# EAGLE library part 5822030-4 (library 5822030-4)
Body Features: Retention Post Location Center | Latch Plating Material Nickel | Connector Profile Standard | Latch Material Brass | Configuration Features: Number of Positions 80 | Module Orientation Vertical | Number of Keys 1 | Number of Rows 1 | Contact Features: Contact Mating Area Plating Material Thickness 200 MICIN | Contact Current Rating (Max) 1 AMP | Contact Mating Area Plating Material Tin | PCB Contact Termination Area Plating Material Tin | Memory Socket Type Memory Card | Contact Base Material Source: Datasheet
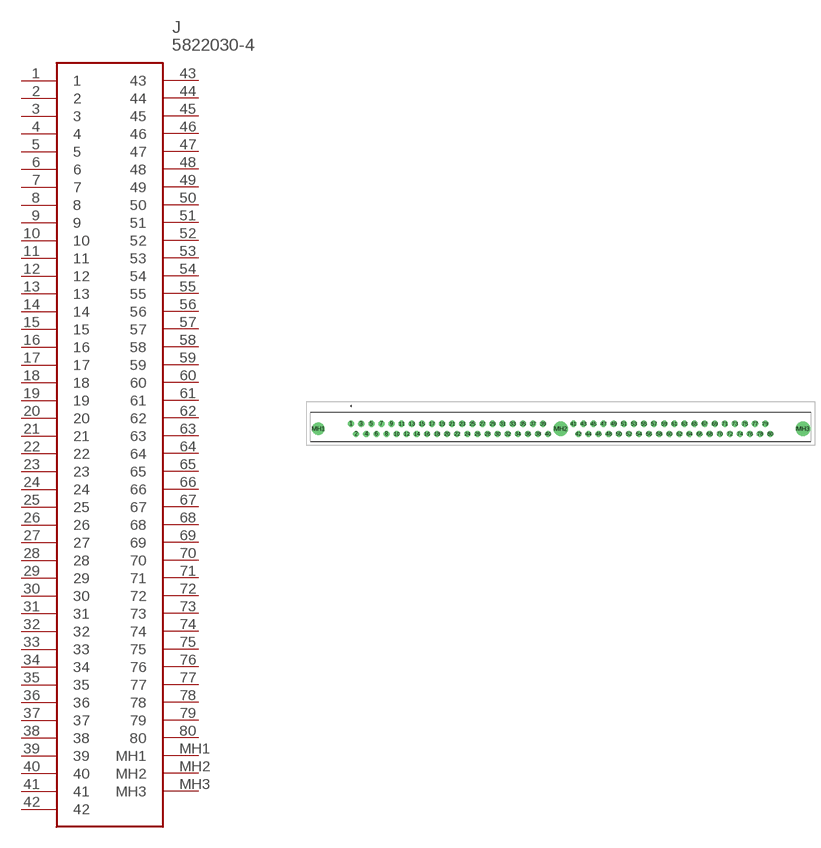
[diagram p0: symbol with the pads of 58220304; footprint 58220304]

Designator prefix J

## 5822030-4 (Description: Body Features: Retention Post Location Center | Latch Plating Material Nickel | Connector Profile Standard | Latch Material Brass | Configuration Features: Number of Positions 80 | Module Orientation Vertical | Number of Keys 1 | Number of Rows 1 | Contact Features: Contact Mating Area Plating Material Thickness 200 MICIN | Contact Current Rating (Max) 1 AMP | Contact Mating Area Plating Material Tin | PCB Contact Termination Area Plating Material Tin | Memory Socket Type Memory Card | Contact Base Material; Height: 14.61mm; Manufacturer_Name: TE Connectivity; Manufacturer_Part_Number: 5822030-4; Mouser_Part_Number: 571-58220304; Mouser_Price-Stock: https://www.mouser.co.uk/ProductDetail/TE-Connectivity/5822030-4?qs=VZ9FDhhp7SlQjd0753bE2g%3D%3D)  [58220304]
1  1
2  2
3  3
4  4
5  5
6  6
7  7
8  8
9  9
10  10
11  11
12  12
13  13
14  14
15  15
16  16
17  17
18  18
19  19
20  20
21  21
22  22
23  23
24  24
25  25
26  26
27  27
28  28
29  29
30  30
31  31
32  32
33  33
34  34
35  35
36  36
37  37
38  38
39  39
40  40
41  41
42  42
43  43
44  44
45  45
46  46
47  47
48  48
49  49
50  50
51  51
52  52
53  53
54  54
55  55
56  56
57  57
58  58
59  59
60  60
61  61
62  62
63  63
64  64
65  65
66  66
67  67
68  68
69  69
70  70
71  71
72  72
73  73
74  74
75  75
76  76
77  77
78  78
79  79
80  80
MH1  MH1
MH2  MH2
MH3  MH3

## Footprint 58220304 (pad centres in mm)
5822030-4-2
drill 1.02 pad 1.53: 1 0,0; 2 1.27,-2.54; 3 2.54,0; 4 3.81,-2.54; 5 5.08,0; 6 6.35,-2.54; 7 7.62,0; 8 8.89,-2.54; 9 10.16,0; 10 11.43,-2.54; 11 12.7,0; 12 13.97,-2.54; 13 15.24,0; 14 16.51,-2.54; 15 17.78,0; 16 19.05,-2.54; 17 20.32,0; 18 21.59,-2.54; 19 22.86,0; 20 24.13,-2.54; 21 25.4,0; 22 26.67,-2.54; 23 27.94,0; 24 29.21,-2.54; 25 30.48,0; 26 31.75,-2.54; 27 33.02,0; 28 34.29,-2.54; 29 35.56,0; 30 36.83,-2.54; 31 38.1,0; 32 39.37,-2.54; 33 40.64,0; 34 41.91,-2.54; 35 43.18,0; 36 44.45,-2.54; 37 45.72,0; 38 46.99,-2.54; 39 48.26,0; 40 49.53,-2.54; 41 55.88,0; 42 57.15,-2.54; 43 58.42,0; 44 59.69,-2.54; 45 60.96,0; 46 62.23,-2.54; 47 63.5,0; 48 64.77,-2.54; 49 66.04,0; 50 67.31,-2.54; 51 68.58,0; 52 69.85,-2.54; 53 71.12,0; 54 72.39,-2.54; 55 73.66,0; 56 74.93,-2.54; 57 76.2,0; 58 77.47,-2.54; 59 78.74,0; 60 80.01,-2.54; 61 81.28,0; 62 82.55,-2.54; 63 83.82,0; 64 85.09,-2.54; 65 86.36,0; 66 87.63,-2.54; 67 88.9,0; 68 90.17,-2.54; 69 91.44,0; 70 92.71,-2.54; 71 93.98,0; 72 95.25,-2.54; 73 96.52,0; 74 97.79,-2.54; 75 99.06,0; 76 100.33,-2.54; 77 101.6,0; 78 102.87,-2.54; 79 104.14,0; 80 105.41,-2.54
drill 2.03 pad 3.045: MH1 -8.26,-1.27
drill 2.44 pad 3.66: MH2 52.7,-1.27; MH3 113.66,-1.27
